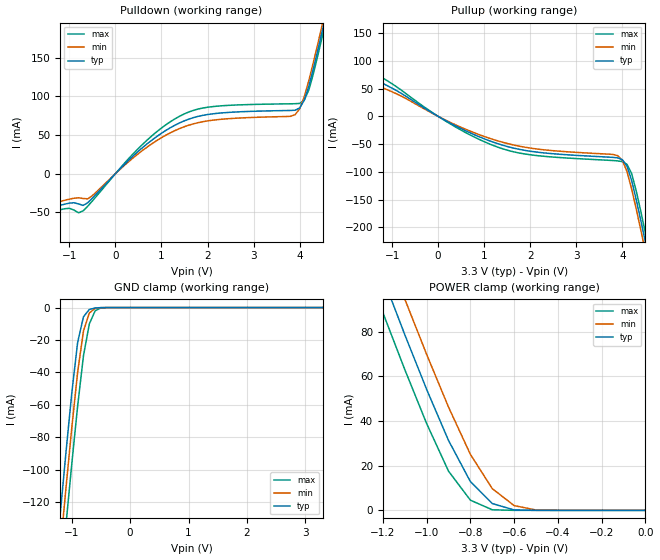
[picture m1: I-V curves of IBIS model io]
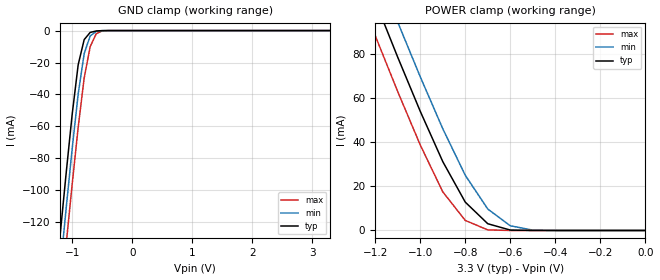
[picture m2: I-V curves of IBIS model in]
[IBIS Ver]   1.1
[File name]   m63z736.ibs
[File Rev]   1.0
[Date]   8/24/98
[Source]   This file originated at Motorola Fast SRAM
[Notes]
1. This I/O model good for MCM63Z736/737
2. Author - Benj Zeller - RA5366
[Disclaimer]   Data is for modeling purposes only and is not guaranteed
[Component]   ZBT RAM
[Manufacturer] Motorola
[Package]
|  RLC Data is subject to change after further study of package
|		typ		min		max
R_pkg		200m		150m		250m
L_pkg		5.5nH		4nH		7nH
C_pkg		2pF		1.5pF		2.5pF
[Pin]		signal_name	model_name	R_pin		L_pin		C_pin
1		DQc		io		NA		NA		NA
2		DCc		io		NA		NA		NA
3		DCc		io		NA		NA		NA
4		VDDQ		POWER		NA		NA		NA
5		VSS		GND		NA		NA		NA
6		DCc		io		NA		NA		NA
7		DCc		io		NA		NA		NA
8		DQc		io		NA		NA		NA
9		DQc		io		NA		NA		NA
10		VSS		GND		NA		NA		NA
11		VDDQ		POWER		NA		NA		NA
12		DQc		io		NA		NA		NA
13		DQc		io		NA		NA		NA
14		VDD		POWER		NA		NA		NA
15		VDD		POWER		NA		NA		NA
16		VDD		POWER		NA		NA		NA
17		VSS		GND		NA		NA		NA
18		DQd		io		NA		NA		NA
19		DQd	 	io		NA		NA		NA
20		VDDQ		POWER		NA		NA		NA
21		VSS		GND		NA		NA		NA
22		DQd		io		NA		NA		NA
23		DQd		io		NA		NA		NA
24		DQd		io		NA		NA		NA
25		DCd		io		NA		NA		NA
26		VSS		GND		NA		NA		NA
27		VDDQ		POWER		NA		NA		NA
28		DCd		io		NA		NA		NA
29		DCd		io		NA		NA		NA
30		DCd		io		NA		NA		NA
31		LBO#		in		NA		NA		NA
32		SA		in		NA		NA		NA
33		SA		in		NA		NA		NA
34		SA		in		NA		NA		NA
35		SA		in		NA		NA		NA
36		SA1		in		NA		NA		NA
37		SA0		in		NA		NA		NA
38		NC		NC		NA		NA		NA
39		NC		NC		NA		NA		NA
40		VSS		GND		NA		NA		NA
41		VDD		POWER		NA		NA		NA
42		NC		NC		NA		NA		NA
43		NC		NC		NA		NA		NA
44		SA		in		NA		NA		NA
45		SA		in		NA		NA		NA
46		SA		in		NA		NA		NA
47		SA		in		NA		NA		NA
48		SA		in		NA		NA		NA
49		SA		in		NA		NA		NA
50		SA		in		NA		NA		NA
51		DQa		io		NA		NA		NA
52		DQa		io		NA		NA		NA
53		DQa		io		NA		NA		NA
54		VDDQ		POWER		NA		NA		NA
55		VSS		GND		NA		NA		NA
56		DQa		io		NA		NA		NA
57		DQa		io		NA		NA		NA
58		DQa		io		NA		NA		NA
59		DQa		io		NA		NA		NA
60		VSS		GND		NA		NA		NA
61		VDDQ		POWER		NA		NA		NA
62		DQa		io		NA		NA		NA
63		DQa		io		NA		NA		NA
64		VSS		GND		NA		NA		NA
65		VDD		POWER		NA		NA		NA
66		VDD		POWER		NA		NA		NA
67		VSS		GND		NA		NA		NA
68		DQb		io		NA		NA		NA
69		DQb		io		NA		NA		NA
70		VDDQ		POWER		NA		NA		NA
71		VSS		GND		NA		NA		NA
72		DQb		io		NA		NA		NA
73		DQb		io		NA		NA		NA
74		DQb		io		NA		NA		NA
75		DQb		io		NA		NA		NA
76		VSS		GND		NA		NA		NA
77		VDDQ		POWER		NA		NA		NA
78		DQb		io		NA		NA		NA
79		DQb		io		NA		NA		NA
80		DQb		io		NA		NA		NA
81		SA		in		NA		NA		NA
82		SA		in		NA		NA		NA
83		NC		NC		NA		NA		NA
84		NC		NC		NA		NA		NA
85		ADV		in		NA		NA		NA
86		G#		in		NA		NA		NA
87		CKE#		in		NA		NA		NA
88		SW#		in		NA		NA		NA
89		CK		in		NA		NA		NA
90		VSS		GND		NA		NA		NA
91		VDD		POWER		NA		NA		NA
92		SE3#		in		NA		NA		NA
93		SBA#		in		NA		NA		NA
94		SBB#		in		NA		NA		NA
95		SBC#		in		NA		NA		NA
96		SBD#		in		NA		NA		NA
97		SE2		in		NA		NA		NA
98		SE1#		in		NA		NA		NA
99		SA		in		NA		NA		NA
100		SA		in		NA		NA		NA
| Models and submodels in the file (2): io (I/O), in (Input)
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| BI-DIRECTIONAL I/O MODEL
[Model]   io
Model_type  I/O
Polarity   Non-Inverting
Enable   Active-Low
|signals  DQa, DQb, DQc, DQd
|Variable   typ   min   max
C_comp   7pF   NA   8pF
|Variable   typ   min   max
[Voltage range]   3.3   3.1  3.6
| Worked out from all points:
|   slope of the pulldown table from 0 to 0.495 V, typ, clamps not added: 17.1 ohm
|   slope of the pullup table from 0 to 0.495 V, typ, clamps not added: 22.6 ohm
|   GND clamp passes 1 mA (typ) near -0.68 V on its own axis
|   POWER clamp passes 1 mA (typ) near -0.63 V on its own axis
|Temp used   50C   100C   0C
|Variable   typ   min   max
|NOTE: All V/I tables should have at least 3 entries.
|   0.0 volts, 2*supply_voltage and -supply_voltage
[Pulldown]
|Volt	Typical		Minimum		Maximum
-3.3V     -73.3mA    -66.9mA    -80.4mA
-1.1V     -39.43mA   -34.43mA   -45.37mA
-700mV    -41.11mA   -32.14mA   -48.09mA
-500mV    -31.7mA    -28.44mA   -35.3mA
600mV     34.3mA     30.61mA    38.6mA
1.6V      70.78mA    62.91mA    80.03mA
3.9V      82.14mA    76.38mA    90.6mA
4.1V      95.09mA    99.58mA    95.41mA
4.2V      113.7mA    120.9mA    108.6mA
4.5V      187.3mA    195.5mA    180.3mA
4.6V      213.8mA    221.8mA    206.9mA
6.6V      818.3mA    815.7mA    823.4mA
[Pullup]
|Volt	Typical		Minimum		Maximum
-3.3V     128.6mA    104.2mA    160.3mA
-1.3V     63.3mA     54.53mA    73.94mA
200mV     -9.267mA   -8.327mA   -10.43mA
1.1V      -43.61mA   -39.12mA   -49.23mA
2V        -62.86mA   -57.16mA   -69.24mA
3.9V      -74.83mA   -70.95mA   -80.32mA
4.1V      -89.65mA   -99.49mA   -86.6mA
4.2V      -115.4mA   -130.9mA   -102.8mA
4.4V      -187.8mA   -205mA     -171.6mA
4.5V      -226.9mA   -244.1mA   -210.7mA
4.6V      -266.8mA   -283.8mA   -250.7mA
6.6V      -1.106A    -1.119A    -1.095A
[GND_clamp]
|Volt	Typical		Minimum		Maximum
-3.3V     -1A        -1.018A    -1.036A
-1.2V     -127.9mA   -149.9mA   -172.5mA
-1.1V     -89.25mA   -111.3mA   -133.8mA
-1V       -52.54mA   -74mA      -96.26mA
-900mV    -21.42mA   -39.77mA   -60.66mA
-800mV    -5.65mA    -14.43mA   -29.67mA
-700mV    -1.151mA   -3.372mA   -10.08mA
-600mV    -259uA     -484.6uA   -1.988mA
-500mV    -23.69uA   -59.55uA   -196.3uA
3.3V      59.55pA    69.04pA    309.5pA
[POWER_clamp]
|Volt	Typical		Minimum		Maximum
-3.3V     705.2mA    714mA      697.1mA
-1.3V     130.4mA    146.3mA    114.8mA
-1.2V     104.3mA    120.2mA    88.55mA
-1.1V     78.73mA    94.65mA    63.09mA
-1V       54.17mA    69.86mA    38.87mA
-900mV    31.32mA    46.25mA    17.57mA
-800mV    12.88mA    25.07mA    4.562mA
-700mV    3.056mA    9.726mA    258.7uA
-600mV    186.1uA    2.13mA     4.238uA
-500mV    5.457uA    152.4uA    62.26nA
0V        69.04pA    309.5pA    59.55pA
[Ramp]
|Variable   typ   min	max
dV/dt_r  1.32/0.30n	NA	NA
dV/dt_f  1.44/0.30n	NA	NA
| STANDARD INPUT MODEL
[Model]   in
Model_type  Input
Polarity   Non-Inverting
|signals  ADV#, G#, CK, SA, SBx#, SE1#, SE2, SE3#, SGW#, SW#
|CKE#, LBO#
|Variable   typ   min   max
C_comp   4pF   NA   5pF
|Variable   typ   min   max
[Voltage range]   3.3   3.1  3.6
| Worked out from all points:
|   GND clamp passes 1 mA (typ) near -0.68 V on its own axis
|   POWER clamp passes 1 mA (typ) near -0.63 V on its own axis
|Temp used   50C   100C   0C
[GND_clamp]
|Volt	Typical		Minimum		Maximum
-3.3V     -1A        -1.018A    -1.036A
-1.2V     -127.9mA   -149.9mA   -172.5mA
-1.1V     -89.25mA   -111.3mA   -133.8mA
-1V       -52.54mA   -74mA      -96.26mA
-900mV    -21.42mA   -39.77mA   -60.66mA
-800mV    -5.65mA    -14.43mA   -29.67mA
-700mV    -1.151mA   -3.372mA   -10.08mA
-600mV    -259uA     -484.6uA   -1.988mA
-500mV    -23.69uA   -59.55uA   -196.3uA
3.3V      59.55pA    69.04pA    309.5pA
[POWER_clamp]
|Volt	Typical		Minimum		Maximum
-3.3V     705.2mA    714mA      697.1mA
-1.3V     130.4mA    146.3mA    114.8mA
-1.2V     104.3mA    120.2mA    88.55mA
-1.1V     78.73mA    94.65mA    63.09mA
-1V       54.17mA    69.86mA    38.87mA
-900mV    31.32mA    46.25mA    17.57mA
-800mV    12.88mA    25.07mA    4.562mA
-700mV    3.056mA    9.726mA    258.7uA
-600mV    186.1uA    2.13mA     4.238uA
-500mV    5.457uA    152.4uA    62.26nA
0V        69.04pA    309.5pA    59.55pA
